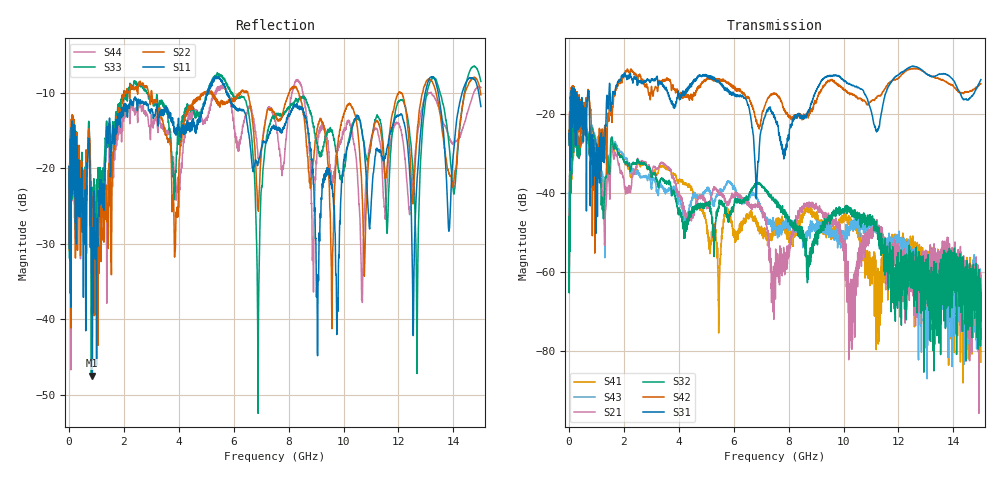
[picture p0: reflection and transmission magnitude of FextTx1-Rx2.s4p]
! FILE: N:\QM 2007\Prüfprotokolle\Highspeed\Konfektionierte Ltg\L45593-D106\D30\8216\0002\Fext\FextTx1-Rx2.s4p
# MHz S RI R 50.00
! FREQ  S11  S12  S13  S14
!  S21  S22  S23  S24
!  S31  S32  S33  S34
!  S41  S42  S43  S44
!  REAL  IMAG  REAL  IMAG  REAL  IMAG  REAL  IMAG
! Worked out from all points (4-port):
!   2999 points, 10 MHz to 15 GHz, reference 50 ohm
!   strongest paths, dB at 10 MHz, 3.755 GHz, 7.505 GHz, 11.26 GHz, 15 GHz:
!     S31: -24.9, -16.7, -21.0, -23.8, -11.3
!     S42: -24.1, -13.1, -14.8, -15.4, -12.4
!     S32: -46.0, -40.6, -42.5, -50.2, -64.4
!     S21: -45.1, -36.2, -58.5, -48.3, -74.0
!     S43: -39.8, -40.4, -47.7, -51.3, -61.1
!     S41: -44.0, -35.9, -48.7, -63.3, -82.8
!   lowest |S11| = -47.5 dB at 855 MHz (marker M1), VSWR 1.01, Z = 49.8 - j0.341 ohm
!   |S11| at or under -10 dB: start of sweep to 5.038 GHz; 5.777 GHz to 12.97 GHz (7.196 GHz wide, 76.8 % of centre); 13.45 GHz to 14.32 GHz (869.5 MHz wide, 6.26 % of centre)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
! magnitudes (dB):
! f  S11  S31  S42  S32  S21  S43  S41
! 10 MHz  -19.8  -24.9  -24.1  -46.0  -45.1  -39.8  -44.0
! 855 MHz  -47.5  -26.3  -50.8  -23.6  -23.6  -23.0  -23.5
! 5.46 GHz  -8.1  -11.6  -11.2  -43.7  -39.8  -39.4  -69.8
! 6.84 GHz  -19.2  -38.0  -21.9  -37.6  -43.0  -41.1  -47.4
! 8.475 GHz  -12.0  -20.4  -20.4  -49.7  -44.5  -51.4  -47.5
! 12.67 GHz  -22.0  -8.1  -8.6  -65.5  -63.7  -57.3  -53.7
! 15 GHz  -11.8  -11.3  -12.4  -64.4  -74.0  -61.1  -82.8
